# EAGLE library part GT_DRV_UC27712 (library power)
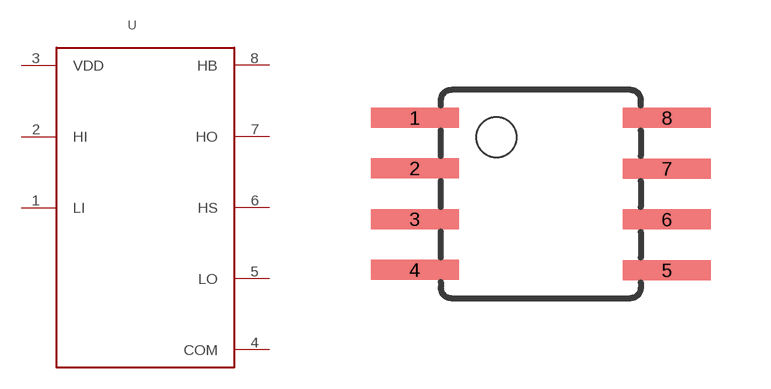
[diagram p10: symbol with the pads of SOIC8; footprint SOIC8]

Designator prefix U

## GT_DRV_UC27712  [SOIC8]
1  LI
2  HI
3  VDD
4  COM
5  LO
6  HS
7  HO
8  HB

## Footprint SOIC8 (pad centres in mm)
Wide Plastic Gull Wing Small Outline Package
smd 2.2 x 0.5: 1 -3.154,1.905; 2 -3.154,0.645; 3 -3.154,-0.625; 4 -3.154,-1.895; 5 3.154,-1.905; 6 3.154,-0.635; 7 3.154,0.635; 8 3.154,1.905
